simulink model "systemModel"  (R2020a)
settings: Solver=VariableStepAuto  StartTime=0.0  StopTime=10.0  RelTol=1e-3
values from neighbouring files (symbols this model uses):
  x0 = [0.2;0.1]    [initParams.m]

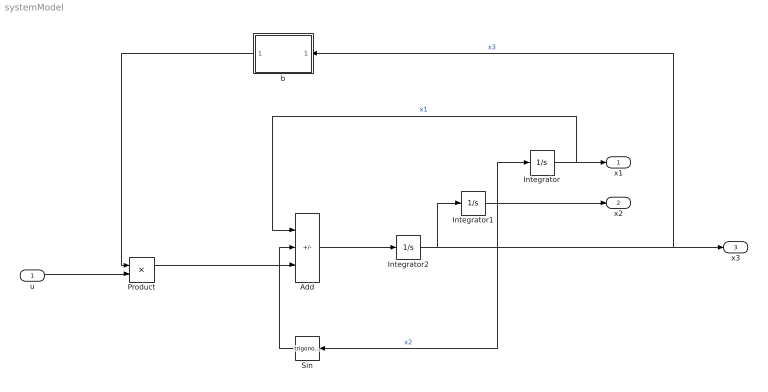
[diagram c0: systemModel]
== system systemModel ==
  u : Inport
  Add : Sum  Inputs=--+
  Integrator : Integrator  InitialCondition=x0(1)
  Integrator1 : Integrator  InitialCondition=x0(2)
  Integrator2 : Integrator  InitialCondition=x0(3)
  Product : Product
  Sin : Trigonometry
  b : MATLAB Function  TreatAsAtomicUnit=on
  x1 : Outport
  x2 : Outport  Port=2
  x3 : Outport  Port=3
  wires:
  Integrator2/1 -> b/1(x3), x3/1, Integrator1/1  "x3"
  u/1 -> Product/2
  b/1(y) -> Product/1
  Sin/1 -> Add/2
  Add/1 -> Integrator2/1
  Integrator1/1 -> x2/1, Sin/1, Integrator/1  "x2"
  Integrator/1 -> Add/1, x1/1  "x1"
  Product/1 -> Add/3

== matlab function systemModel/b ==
function y = fcn(x3)

y = exp(-x3)+1;
